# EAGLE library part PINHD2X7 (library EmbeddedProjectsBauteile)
PIN HEADER 2 x 7 polig
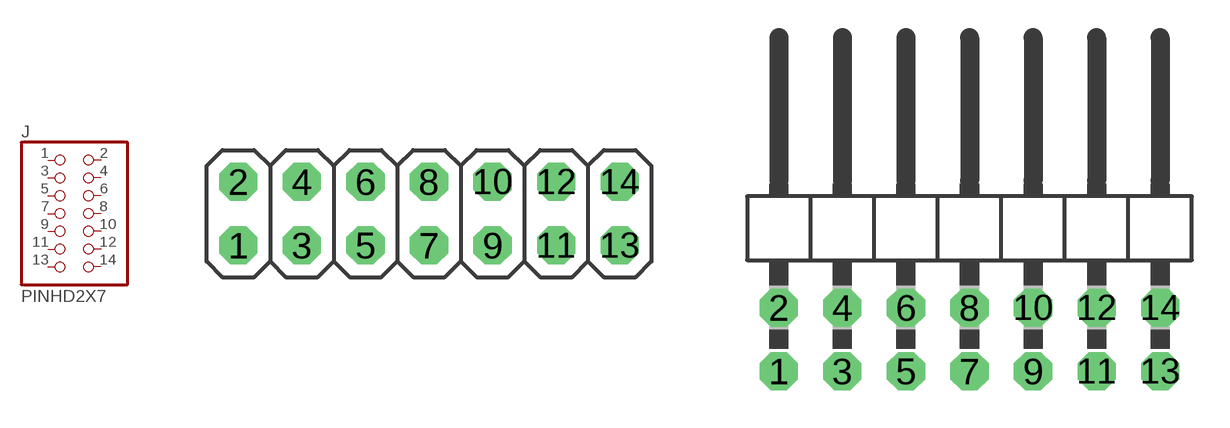
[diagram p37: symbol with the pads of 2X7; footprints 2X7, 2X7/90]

Designator prefix J

## PINHD2X7STEHEND (EP: 400414)  [2X7]
1  1  pas
2  2  pas
3  3  pas
4  4  pas
5  5  pas
6  6  pas
7  7  pas
8  8  pas
9  9  pas
10  10  pas
11  11  pas
12  12  pas
13  13  pas
14  14  pas

## PINHD2X7LIEGEND  [2X7/90]
Pads as for 2X7

## Footprint 2X7 (pad centres in mm)
drill 1.016 octagon: 1 -6.35,-1.27; 2 -6.35,1.27; 3 -3.81,-1.27; 4 -3.81,1.27; 5 -1.27,-1.27; 6 -1.27,1.27; 7 1.27,-1.27; 8 1.27,1.27; 9 3.81,-1.27; 10 3.81,1.27; 11 6.35,-1.27; 12 6.35,1.27; 13 8.89,-1.27; 14 8.89,1.27

## Footprint 2X7/90 (pad centres in mm)
drill 1.016 octagon: 1 -7.62,-3.81; 2 -7.62,-1.27; 3 -5.08,-3.81; 4 -5.08,-1.27; 5 -2.54,-3.81; 6 -2.54,-1.27; 7 0,-3.81; 8 0,-1.27; 9 2.54,-3.81; 10 2.54,-1.27; 11 5.08,-3.81; 12 5.08,-1.27; 13 7.62,-3.81; 14 7.62,-1.27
